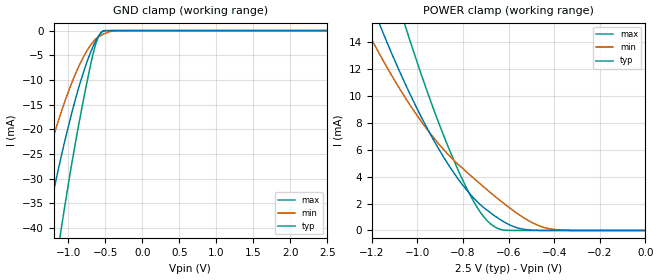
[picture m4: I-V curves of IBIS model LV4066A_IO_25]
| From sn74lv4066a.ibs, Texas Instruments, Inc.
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[Model]   LV4066A_IO_25
Model_type  Terminator
| variable   typ   min   max
C_comp   7.02pF   5.93pF   7.66pF
| C_tri-state   7.02pF   5.93pF   7.66pF
[Temperature Range]   40   100   -40
| Ambient temperature   25   85   -40
[Voltage range]   2.5   2.3   2.7
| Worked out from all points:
|   GND clamp passes 1 mA (typ) near -0.59 V on its own axis
|   POWER clamp passes 1 mA (typ) near -0.65 V on its own axis
[GND Clamp]
| LV4066A_IO_25
|   Voltage   I(typ)   I(min)   I(max)
-2.5V     -152.5mA   -106.7mA   -221mA
-1.55V    -60.17mA   -40.6mA    -90.41mA
-1.32V    -41.55mA   -27.53mA   -63.64mA
-1.29V    -39.27mA   -25.95mA   -60.34mA
-1.105V   -26.14mA   -16.92mA   -41.13mA
-1.09V    -25.15mA   -16.25mA   -39.66mA
-895mV    -13.45mA   -8.499mA   -22.01mA
-705mV    -4.652mA   -3.093mA   -7.403mA
-620mV    -1.842mA   -1.592mA   -2.332mA
-535mV    -192.3uA   -789.4uA   -97.35uA
-310mV    -62.21nA   -7.607uA   -2.678nA
2.5V      62.15pA    169.1nA    46.93pA
[POWER Clamp]
| LV4066A_IO_25
|   Voltage   I(typ)   I(min)   I(max)
-2.5V     97.54mA    76.04mA    131mA
-1.23V    18.1mA     15.16mA    25.44mA
-1.15V    14.67mA    12.63mA    20.62mA
-1.05V    10.77mA    9.783mA    15.03mA
-930mV    6.749mA    6.918mA    9.058mA
-830mV    4.03mA     5.053mA    4.809mA
-745mV    2.264mA    3.763mA    1.909mA
-680mV    1.318mA    2.821mA    497.3uA
-635mV    787.2uA    2.196mA    75.78uA
-565mV    208.7uA    1.3mA      2.305uA
-435mV    2.666uA    180.2uA    12.57nA
-31.15fV  62.15pA    582.8pA    62.13pA
